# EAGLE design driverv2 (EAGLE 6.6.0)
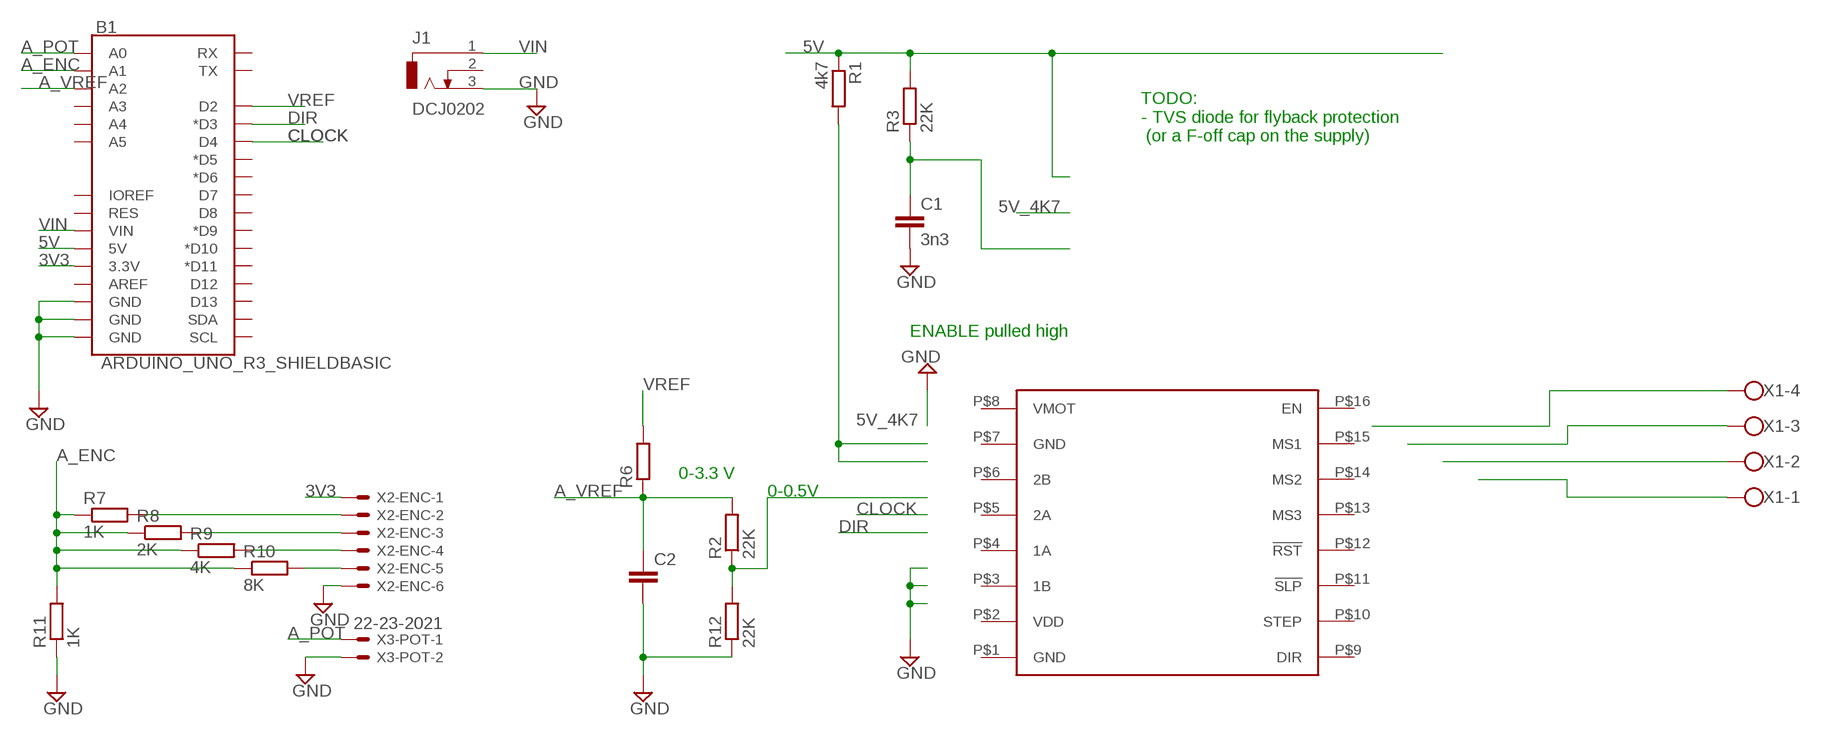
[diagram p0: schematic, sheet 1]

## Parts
B1  ARDUINO_UNO_R3_SHIELDBASIC  [UNO_R3_SHIELD]
C1  3n3  C-EU050-030X075  [C050-030X075]
C2  C-EU050-030X075  [C050-030X075]
J1  DCJ0202  [DCJ0202]
R1  4k7  R-EU_0309/V  [0309V]
R2  22K  R-EU_0309/V  [0309V]
R3  22K  R-EU_0309/V  [0309V]
R6  R-EU_0309/V  [0309V]
R7  1K  R-EU_0309/V  [0309V]
R8  2K  R-EU_0309/V  [0309V]
R9  4K  R-EU_0309/V  [0309V]
R10  8K  R-EU_0309/V  [0309V]
R11  1K  R-EU_0309/V  [0309V]
R12  22K  R-EU_0309/V  [0309V]
U$1  POLOLU-2980  [POLOLU-2980]
X1  W237-4  [W237-4]
X2-ENC  22-23-2061  [22-23-2061]
X3-POT  22-23-2021  [22-23-2021]

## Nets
3V3: B1.3.3V X2-ENC.1
5V: B1.5V R1.1 R3.2
5V_4K7: R1.2
A_ENC: B1.A1 R7.1 R8.1 R9.1 R10.1 R11.2
A_POT: B1.A0 X3-POT.1
A_VREF: B1.A2 C2.1 R2.2 R6.1
CLOCK: B1.D4
DIR: B1.D3(*D3)
GND [drive]: B1.GND@0(GND) B1.GND@1(GND) B1.GND@2(GND) C1.2 C2.2 J1.3 R11.1 R12.1 X2-ENC.6 X3-POT.2
N$1: R2.1 R12.2
N$2: C1.1 R3.1
N$13 [drive]: X1.4
N$14 [drive]: X1.3
N$15 [drive]: X1.2
N$16 [drive]: X1.1
N$20: R7.2 X2-ENC.2
N$21: R8.2 X2-ENC.3
N$22: R9.2 X2-ENC.4
N$23: R10.2 X2-ENC.5
VIN [drive]: B1.VIN J1.1
VREF: B1.D2 R6.2
Unconnected: B1.A3 B1.A4 B1.A5 B1.AREF B1.D5(*D5) B1.D6(*D6) B1.D7 B1.D8 B1.D9(*D9) B1.D10(*D10) B1.D11(*D11) B1.D12 B1.D13 B1.IOREF B1.RES B1.RX B1.SCL B1.SDA B1.TX J1.2 U$1.P$1(GND) U$1.P$2(VDD) U$1.P$3(1B) U$1.P$4(1A) U$1.P$5(2A) U$1.P$6(2B) U$1.P$7(GND) U$1.P$8(VMOT) U$1.P$9(DIR) U$1.P$10(STEP) U$1.P$11(!SLP) U$1.P$12(!RST) U$1.P$13(MS3) U$1.P$14(MS2) U$1.P$15(MS1) U$1.P$16(EN)

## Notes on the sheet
- TODO:
  - TVS diode for flyback protection 
   (or a F-off cap on the supply)
- ENABLE pulled high
- 0-3.3 V
- 0-0.5V

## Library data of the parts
B1 = SparkFun-Boards:ARDUINO_UNO_R3_SHIELD: Arduino R3 Shield Footprint Shield form compatible with the Arduino Uno R3. SparkFun Products: MG2639 Cellular Shield MIDI Shield R3 Stackable Headers Kit
C1 C2 = resistor:C-EU: CAPACITOR, European symbol
J1 = con-jack:DCJ0202: DC POWER JACK Source: DCJ0202.pdf; OC_FARNELL: unknown; OC_NEWARK: unknown
R1-R3 R6-R12 = rcl:R-EU_: RESISTOR, European symbol
U$1 = lib:POLOLU-2980
X1 = con-wago-500:W237-4: WAGO SCREW CLAMP; OC_FARNELL: unknown; OC_NEWARK: unknown
X2-ENC = con-molex:22-23-2061: .100" (2.54mm) Center Header - 6 Pin; MF: MOLEX; MPN: 22-23-2061; OC_FARNELL: 1462922; OC_NEWARK: 27C1933
X3-POT = con-molex:22-23-2021: .100" (2.54mm) Center Header - 2 Pin; MF: MOLEX; MPN: 22-23-2021; OC_FARNELL: 1462926; OC_NEWARK: 25C3832

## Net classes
0 default: clearance 0.203 mm
1 drive: width 0.813 mm, drill 1.016 mm, clearance 0.305 mm to class 0, clearance 0.203 mm

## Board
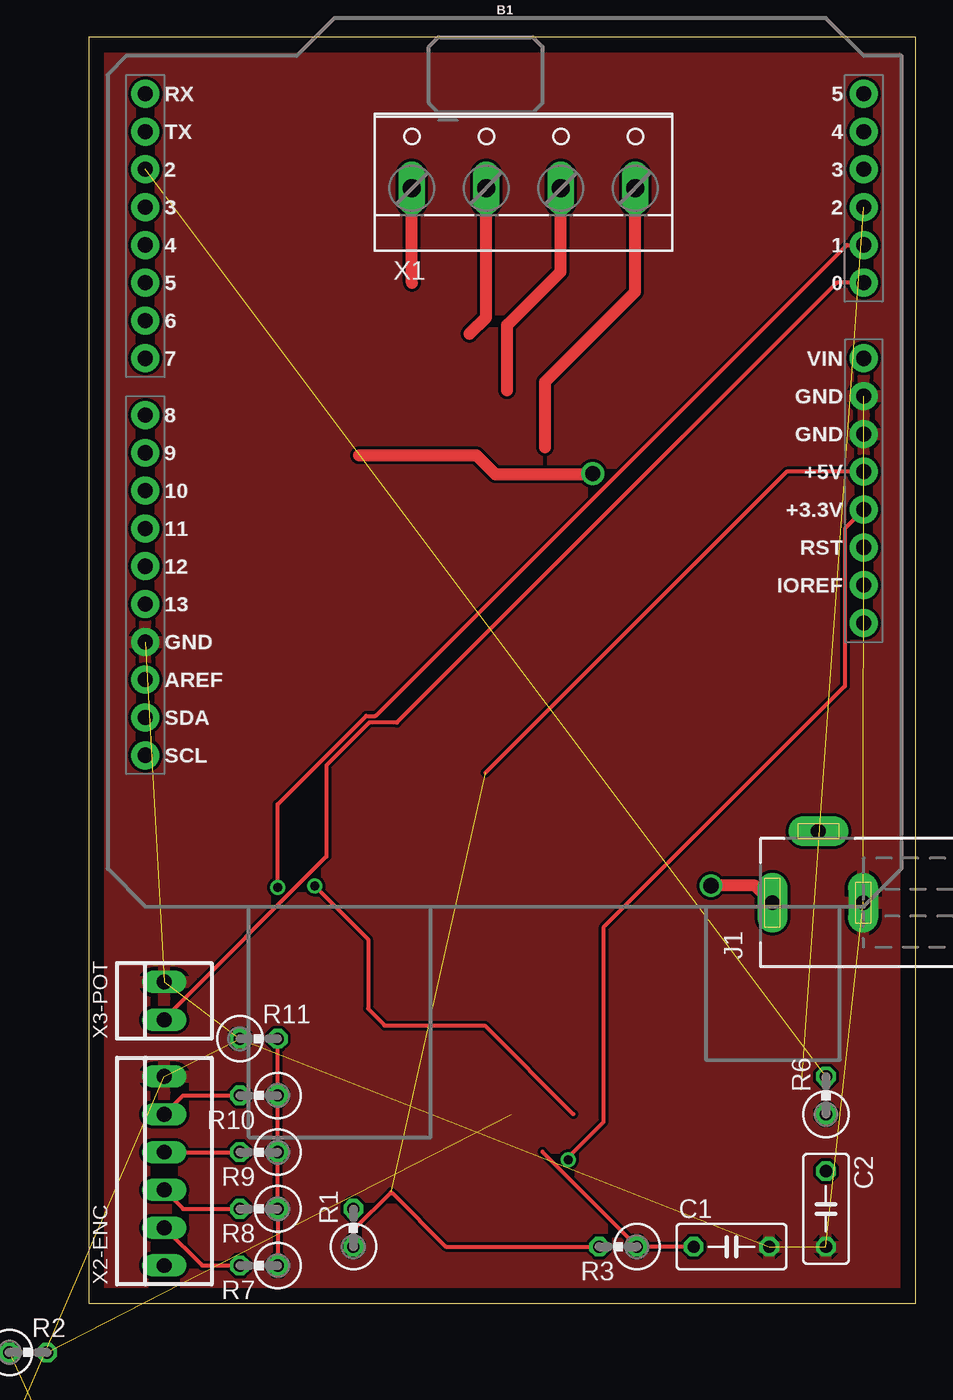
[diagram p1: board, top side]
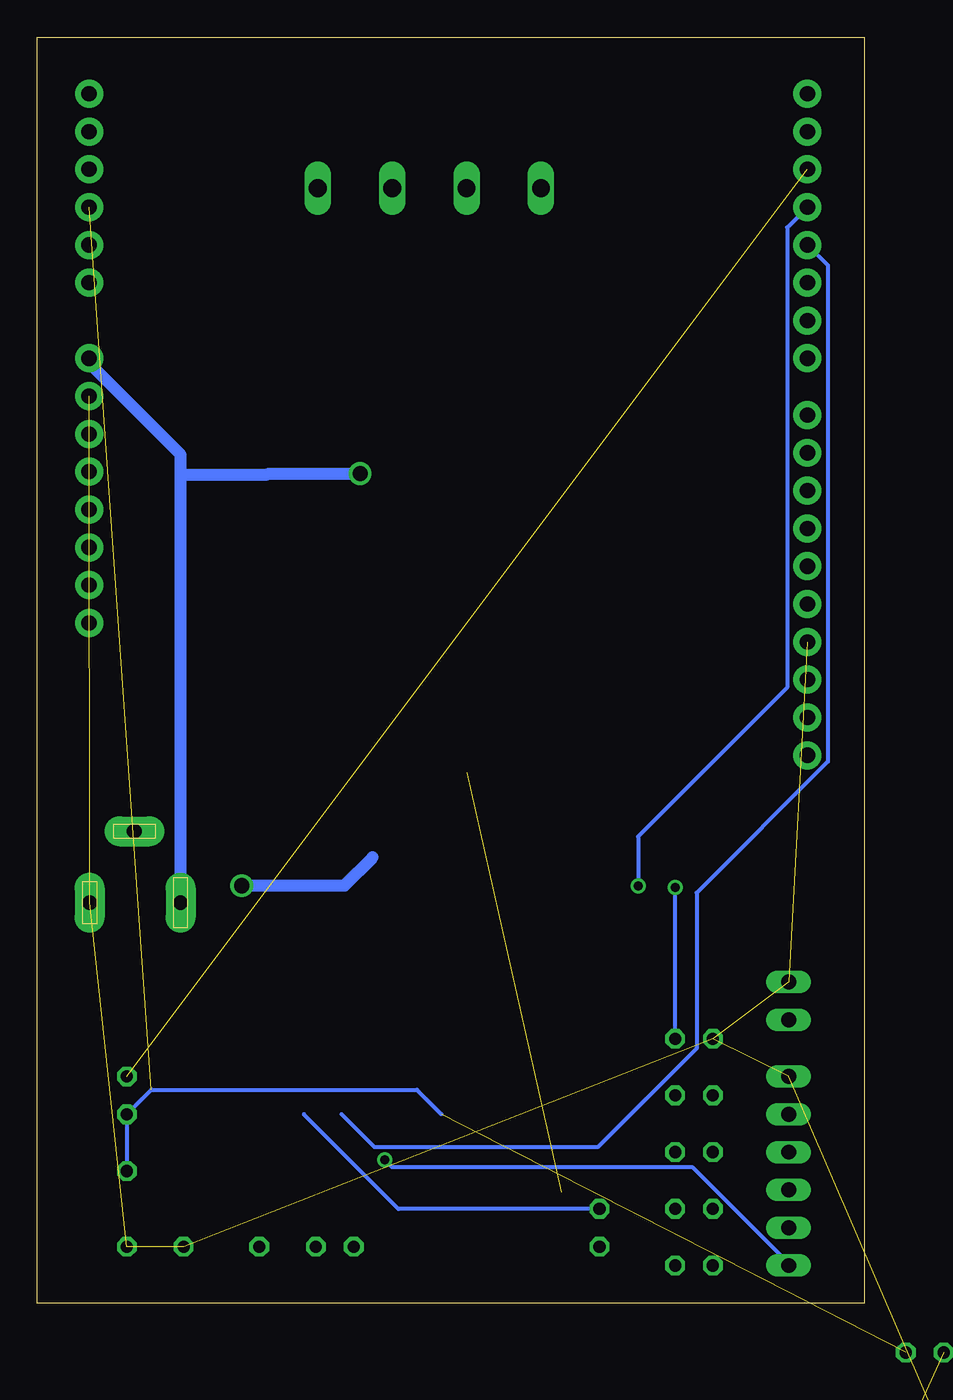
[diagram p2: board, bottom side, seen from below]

Size 55.55 x 85.08 mm. Coordinates in mm from the lower left corner, seen from the top.
Outline: 0,0 55.55,0 55.55,85.08 0,85.08 0,0
Copper layers (1*16): Top 0.035mm / dielectric 1.5mm / Bottom 0.035mm
Design rules "default": minimum track width 10mil, minimum drill 24mil, track to track 8mil, track to pad 8mil, pad to pad 8mil, via to via 8mil, smd to smd 8mil, copper to edge 40mil, drill to drill 8mil, minimum pad ring 10mil, minimum via ring 8mil, stop-mask expansion 4mil, vias tented up to drill 0mil, thermal gap 10mil

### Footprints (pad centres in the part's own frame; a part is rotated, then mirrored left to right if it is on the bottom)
UNO_R3_SHIELD = drill 1.016 pad 1.88: 3.3V 24.13,-2.54; 5V 24.13,0; A0 24.13,12.7; A1 24.13,15.24; A2 24.13,17.78; A3 24.13,20.32; A4 24.13,22.86; A5 24.13,25.4; AREF -24.13,-13.97; D2 -24.13,20.32; D3 -24.13,17.78; D4 -24.13,15.24; D5 -24.13,12.7; D6 -24.13,10.16; D7 -24.13,7.62; D8 -24.13,3.81; D9 -24.13,1.27; D10 -24.13,-1.27; D11 -24.13,-3.81; D12 -24.13,-6.35; D13 -24.13,-8.89; GND@0 24.13,2.54; GND@1 24.13,5.08; GND@2 -24.13,-11.43; IOREF 24.13,-7.62; NC 24.13,-10.16; RES 24.13,-5.08; RX -24.13,25.4; SCL -24.13,-19.05; SDA -24.13,-16.51; TX -24.13,22.86; VIN 24.13,7.62
C050-030X075 = drill 0.813 octagon: 1 -2.54,0; 2 2.54,0
DCJ0202 = drill 1 pad 2 long: 1 0,3.1; 2 4.8,0; 3 0,-3
0309V = drill 0.813 octagon: 1 -1.27,0; 2 1.27,0
POLOLU-2980 = drill 0.8 square: P$1 6.35,-8.89 | drill 0.8: P$2 6.35,-6.35; P$3 6.35,-3.81; P$4 6.35,-1.27; P$5 6.35,1.27; P$6 6.35,3.81; P$7 6.35,6.35; P$8 6.35,8.89; P$9 -6.35,-8.89; P$10 -6.35,-6.35; P$11 -6.35,-3.81; P$12 -6.35,-1.27; P$13 -6.35,1.27; P$14 -6.35,3.81; P$15 -6.35,6.35; P$16 -6.35,8.89
W237-4 = drill 1.194 long: 1 -7.5,-1.27; 2 -2.5,-1.27; 3 2.5,-1.27; 4 7.5,-1.27
22-23-2061 = drill 1 long: 1 -6.35,0; 2 -3.81,0; 3 -1.27,0; 4 1.27,0; 5 3.81,0; 6 6.35,0
22-23-2021 = drill 1 long: 1 -1.27,0; 2 1.27,0

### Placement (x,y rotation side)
B1  27.94,55.88 0 top
C1  43.18,3.81 0 top
C2  49.53,6.35 270 top
J1  49.02,26.92 90 top
R1  17.78,5.08 90 top
R2  not placed on the board
R3  35.56,3.81 180 top
R6  49.53,13.97 90 top
R7  11.43,2.54 180 top
R8  11.43,6.35 180 top
R9  11.43,10.16 180 top
R10  11.43,13.97 180 top
R11  11.43,17.78 0 top
R12  not placed on the board
U$1  not placed on the board
X1  29.21,76.2 0 top
X2-ENC  5.08,8.89 90 top
X3-POT  5.08,20.32 90 top

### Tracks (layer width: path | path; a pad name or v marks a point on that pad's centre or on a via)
3V3  (via drill 0.61)
  Top 0.254: v32.21,9.65 32.21,9.8 34.57,12.17 34.57,25.25 50.8,41.48 50.8,52.07 B1.3.3V
  Bottom 0.254: X2-ENC.1 5.08,2.69 11.56,9.17 31.73,9.17 v32.21,9.65
5V  (1 unrouted)
  Top 0.254: R1.1 17.78,4.93 20.32,7.47 20.42,7.39 24,3.81 R3.2 | 26.67,35.66 46.89,55.88 B1.5V
5V_4K7
  Bottom 0.254: 37.64,12.7 31.29,6.35 R1.2
A_ENC  (via drill 0.61)
  Top 0.254: R7.1 R8.1 R9.1 R10.1 R11.2 | B1.A1 50.93,71.12 19.28,39.47 18.64,39.47 12.7,33.53 v12.7,27.94
  Bottom 0.254: R11.2 v12.7,27.94
A_POT
  Top 0.254: X3-POT.1 5.08,19.13 15.98,30.02 15.98,36.14 18.85,39.01 20.7,39.01 50.27,68.58 B1.A0
A_VREF  (2 unrouted)
  Bottom 0.254: 28.4,12.7 30.05,14.35 47.88,14.35 R6.1 C2.1
CLOCK
  Bottom 0.254: 35.1,12.7 32.89,10.49 17.91,10.49 11.25,17.14 11.25,27.58 2.44,36.4 2.44,69.75 B1.D4
DIR  (via drill 0.61)
  Top 0.254: 32.56,12.7 26.59,18.67 19.89,18.67 18.77,19.79 18.77,24.46 v15.19,28.04
  Bottom 0.254: v15.19,28.04 15.19,31.37 5.18,41.38 5.18,72.29 B1.D3
GND  (9 unrouted)
  pour Top: 0,85.09 0,0 55.88,0 55.88,85.09
N$1  (1 unrouted)
N$2
  Top 0.254: C1.1 R3.1 36.75,3.91 30.48,10.19
N$13
  Top 0.813: 30.66,57.53 30.66,61.92 36.7,67.97 X1.4
N$14
  Top 0.813: 28.12,61.34 28.12,65.73 31.7,69.32 31.7,74.93 X1.3
N$15
  Top 0.813: 25.58,65.15 26.7,66.27 26.7,74.93 X1.2
N$16
  Top 0.813: 21.72,68.58 X1.1
N$20
  Top 0.254: R7.2 7.62,2.54 X2-ENC.2
N$21
  Top 0.254: R8.2 6.35,6.35 X2-ENC.3
N$22
  Top 0.254: X2-ENC.4 R9.2
N$23
  Top 0.254: R10.2 6.35,13.97 X2-ENC.5
VIN  (via drill 1.02)
  Top 0.813: v41.81,28.07 44.76,28.07 45.9,26.92 J1.1 | 18.16,56.97 26.06,56.97 27.33,55.7 33.81,55.7 v33.86,55.75
  Bottom 0.813: 33.02,29.97 34.93,28.07 v41.81,28.07 | B1.VIN 52.07,63.17 45.92,57.02 45.92,55.7 | 45.92,55.7 J1.1 | v33.86,55.75 40.03,55.75 40.08,55.7 45.92,55.7
VREF  (1 unrouted)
